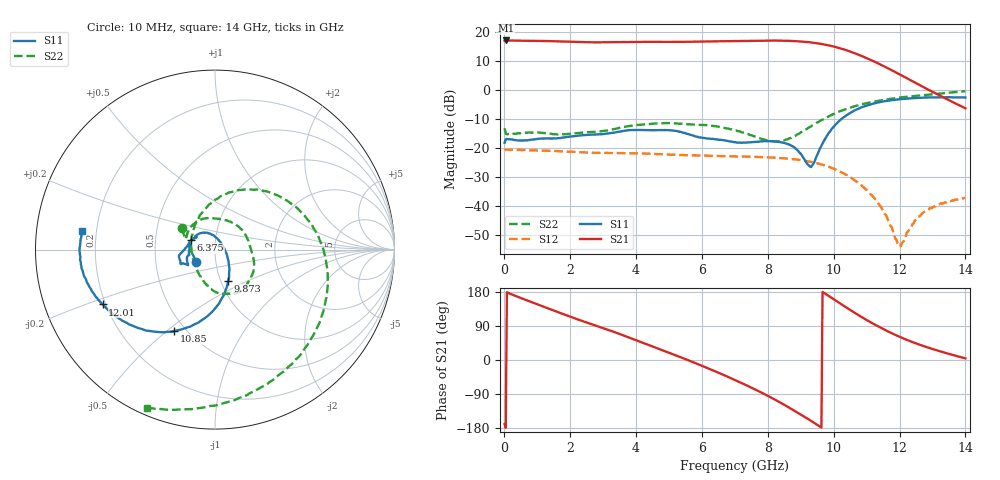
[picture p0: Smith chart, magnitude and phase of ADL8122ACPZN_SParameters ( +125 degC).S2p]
! "Analog Devices, Inc."
! Device:	ADL8122ACPZN
! Description:	"10 kHz to 10 GHz, Wideband, Low Noise Amplifier"
! Conditions:	Vdd = 5.0 V
!		IDQ = 95 mA
!		Pin = -25 dBm
!		Operating Temperature = +25 C (at package bottom)
! Product validation unit SN1 soldered down to Evaluation Board as shown on ADL8122-EVALZ User Guide. Board loss de-embedded from S21 magnitude.  All other RF measurements reference to RF coaxial connector.
! Frequency (GHz)	S11_Mag (dB)	S11_Phase (deg)	S21_Mag (dB)	S21_Phase (deg)	S12_Mag (dB)	S12_Phase (deg)	S22_Mag (dB)	S22_Phase (deg)
#  GHZ  S  DB  R 50
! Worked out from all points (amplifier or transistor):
!   401 points, 10 MHz to 14 GHz, reference 50 ohm
!   highest |S21| = 17.2 dB at 44.98 MHz (marker M1)
!   |S21| within 3 dB of that: start of sweep to 10.28 GHz
!   unconditionally stable (mu >= 1): start of sweep to end of sweep
!   at 2.318 GHz: K = 1.13, MAG = 16.8 dB, |S12| = -21.4 dB
!   at 7.005 GHz: K = 1.17, MAG = 17.4 dB, |S12| = -22.8 dB
!   at 14 GHz: K = 2.19, MAG = 9.3 dB, |S12| = -37.2 dB
!   S11 on the Smith chart (normalised r, x): 10 MHz: 0.80, -0.11; 6.375 GHz: 0.76, +0.08; 9.873 GHz: 1.08, -0.39; 10.85 GHz: 0.43, -0.53; 12.01 GHz: 0.19, -0.22; 14 GHz: 0.14, +0.07
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0.01  -18.12 -147.2  17.02 -169.2  -20.79 9.6  -13.14 147.2
0.044975  -16.98 177.0  17.16 -178.9  -20.46 1.4  -15.01 159.6
0.2898  -17.17 169.1  17.11 170.8  -20.57 -7.3  -15.01 153.6
1.19915  -16.68 -172.2  16.97 140.6  -20.87 -30.8  -14.77 107.9
1.793725  -16.34 -167.8  16.82 121.1  -21.12 -46.1  -15.21 75.4
2.353325  -15.61 -160.2  16.60 103.3  -21.43 -60.2  -14.69 39.9
3.57745  -14.13 -156.7  16.63 66.3  -21.72 -90.4  -12.83 -18.2
4.69665  -13.78 -166.0  16.67 29.2  -22.07 -122.6  -11.43 -53.8
5.571025  -15.11 -178.3  16.70 -0.1  -22.43 -148.1  -11.79 -72.4
6.37545  -16.90 158.1  16.84 -28.8  -22.67 -172.6  -12.41 -87.5
7.005  -17.95 148.7  16.96 -52.8  -22.84 167.6  -13.83 -103.0
7.669525  -17.79 146.7  17.08 -80.0  -23.03 145.3  -16.26 -129.1
8.229125  -17.71 141.7  17.13 -105.0  -23.30 125.3  -17.69 -167.8
8.75375  -19.37 118.8  16.97 -130.9  -23.78 104.2  -16.15 143.0
9.348325  -25.98 12.4  16.42 -162.5  -24.85 78.7  -12.20 99.5
9.87295  -14.49 -67.1  15.41 167.8  -26.48 53.8  -8.89 67.7
10.3626  -8.87 -94.6  13.88 139.8  -29.12 30.6  -6.56 38.3
10.85225  -5.89 -116.6  11.79 113.2  -32.90 7.0  -4.88 10.0
11.69165  -3.56 -145.5  7.31 73.5  -45.69 -42.9  -3.04 -33.4
12.00642  -3.14 -154.0  5.42 61.0  -53.31 -127.0  -2.58 -47.6
12.8808  -2.53 -171.0  0.12 32.5  -41.25 143.3  -1.52 -81.1
14  -2.52 172.2  -6.25 4.2  -37.19 118.8  -0.34 -113.3
